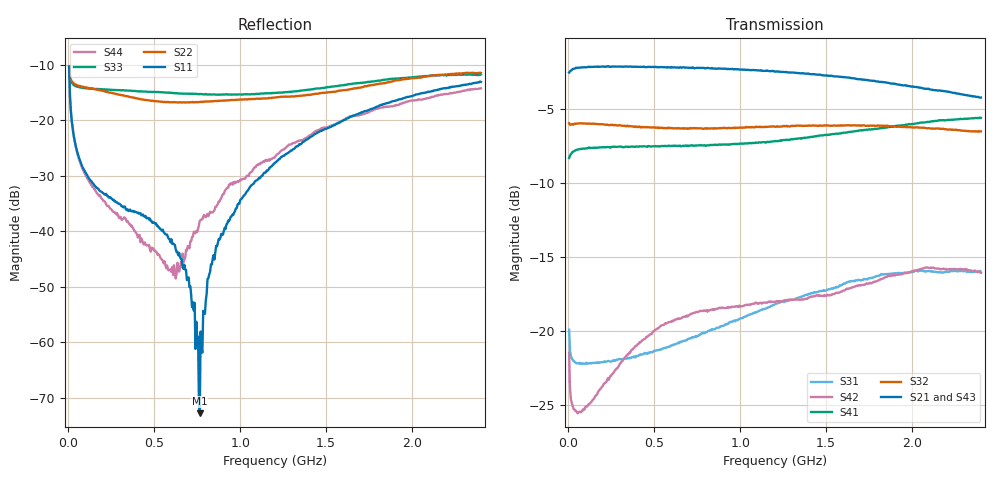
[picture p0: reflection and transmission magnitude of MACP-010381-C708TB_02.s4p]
!Agilent Technologies,E5071B,JP1KK00267,A.09.10
!Date: Mon Mar 23 11:04:21 2020
!Data & Calibration Information:
!DD.  Test Board PCB PT-0014848.  Pin Port mapping: Port1 – pin1, Port1 – pin2, Port3 – pin4, Port4 – pin5
!Freq	S11:SOLT4(ON)	S12:SOLT4(ON)	S13:SOLT4(ON)	S14:SOLT4(ON)
!	S21:SOLT4(ON)	S22:SOLT4(ON)	S23:SOLT4(ON)	S24:SOLT4(ON)
!	S31:SOLT4(ON)	S32:SOLT4(ON)	S33:SOLT4(ON)	S34:SOLT4(ON)
!	S41:SOLT4(ON)	S42:SOLT4(ON)	S43:SOLT4(ON)	S44:SOLT4(ON)
# Hz S MA R 75
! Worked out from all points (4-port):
!   480 points, 5 MHz to 2.4 GHz, reference 75 ohm
!   strongest paths, dB at 5 MHz, 605 MHz, 1.205 GHz, 1.805 GHz, 2.4 GHz:
!     S21: -2.5, -2.2, -2.5, -3.2, -4.2
!     S43: -2.6, -2.2, -2.5, -3.2, -4.1
!     S32: -6.0, -6.3, -6.2, -6.1, -6.5
!     S41: -8.3, -7.5, -7.2, -6.3, -5.6
!     S42: -21.5, -19.3, -18.0, -16.6, -16.1
!     S31: -19.9, -21.0, -18.2, -16.3, -16.0
!   lowest |S11| = -72.8 dB at 765 MHz (marker M1), VSWR 1.00, Z = 75 + j0.0335 ohm
!   |S11| at or under -10 dB: start of sweep to end of sweep
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5000000  0.3029 111.0  0.7434 15.4  0.08269 153.9  0.382 25.8
         0.746 15.3  0.3064 143.5  0.5062 -171.9  0.1024 165.2
         0.101 164.7  0.503 -171.9  0.296 143.9  0.7432 15.4
         0.3838 25.9  0.08445 154.6  0.7386 15.6  0.3046 111.3
2.35e8  0.02013 111.1  0.7826 -6.4  0.05428 155.8  0.4153 -0.5
        0.7837 -6.6  0.1782 161.6  0.5029 163.8  0.08057 157.9
        0.07923 160.8  0.4959 163.4  0.1881 166.1  0.7762 -6.6
        0.4177 -0.5  0.06844 175.7  0.7769 -6.5  0.01684 123.3
6.1e8  0.007728 90.9  0.7787 -19.0  0.07379 123.4  0.4225 -4.3
       0.7759 -18.8  0.1448 158.1  0.4934 139.1  0.09369 128.8
       0.08993 133.5  0.4826 138.6  0.1756 156.6  0.7767 -19.1
       0.4215 -4.4  0.1079 133.7  0.7726 -18.9  0.004023 -158.3
7.65e8  0.0002287 102.2  0.7742 -24.0  0.08528 112.1  0.4227 -5.3
        0.7729 -23.9  0.1457 158.9  0.4924 129.2  0.1027 117.6
        0.09734 122.4  0.4835 129.0  0.172 155.8  0.7719 -24.2
        0.4236 -5.5  0.1169 116.2  0.7682 -23.9  0.01241 -108.4
8.65e8  0.007296 -99.7  0.7701 -27.4  0.09382 105.7  0.4263 -6.1
        0.7683 -27.3  0.1489 158.3  0.4902 122.8  0.1084 110.0
        0.1026 115.4  0.4835 122.7  0.1696 157.0  0.767 -27.5
        0.4251 -6.3  0.1188 106.4  0.7651 -27.3  0.01706 -104.7
1.08e9  0.02693 -106.5  0.7574 -34.5  0.1132 91.9  0.4342 -7.7
        0.7605 -34.5  0.1549 156.5  0.4898 109.0  0.1201 94.4
        0.1153 100.3  0.487 109.1  0.1717 161.2  0.7554 -34.4
        0.4311 -7.7  0.1239 88.3  0.7569 -34.4  0.03694 -105.5
2.4e9  0.2212 -150.1  0.6123 -79.4  0.159 9.9  0.5192 -26.4
       0.614 -79.6  0.2661 137.0  0.473 24.2  0.1506 -4.5
       0.1582 8.2  0.4722 24.7  0.2584 144.4  0.6268 -77.9
       0.5244 -26.5  0.1571 -1.0  0.6233 -78.2  0.1934 -138.6
